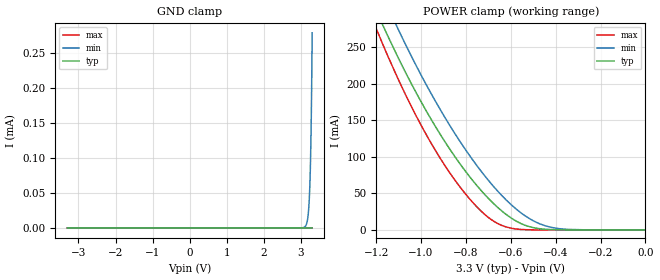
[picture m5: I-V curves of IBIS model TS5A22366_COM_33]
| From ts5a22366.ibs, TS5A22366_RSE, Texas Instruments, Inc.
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[Model]   TS5A22366_COM_33
Model_type  Terminator
| variable   typ   min   max
C_comp   111.30pF   73.64pF   137.43pF
| C_tri-state   111.30pF   73.64pF   137.43pF
[Temperature Range]   40   100   -40
| Ambient temperature   25   85   -40
[Voltage range]   3.3   3   3.6
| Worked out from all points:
|   POWER clamp passes 1 mA (typ) near -0.45 V on its own axis
[GND Clamp]
| TS5A22366_COM_33
|   Voltage   I(typ)   I(min)   I(max)
-3.3V     -7.249nA   -333.8nA   -3.915nA
3.1V      3.718nA    1.468uA    3.133nA
3.15V     3.782nA    5.921uA    3.187nA
3.185V    3.83nA     15.41uA    3.225nA
3.21V     3.87nA     29.93uA    3.251nA
3.235V    3.925nA    57.05uA    3.278nA
3.255V    3.995nA    94.24uA    3.3nA
3.27V     4.079nA    136.2uA    3.316nA
3.28V     4.162nA    173.4uA    3.327nA
3.285V    4.215nA    195.4uA    3.332nA
3.295V    4.353nA    247.6uA    3.343nA
3.3V      4.444nA    278.4uA    3.348nA
[POWER Clamp]
| TS5A22366_COM_33
|   Voltage   I(typ)   I(min)   I(max)
-3.3V     2.841A     2.858A     3.14A
-1.21V    307.7mA    348.5mA    283.5mA
-1.19V    293.8mA    334.3mA    268.5mA
-1.165V   276.8mA    316.9mA    250.3mA
-1.105V   237.9mA    276.9mA    208.7mA
-995mV    173mA      209.4mA    140.7mA
-870mV    109.8mA    142.2mA    77.4mA
-770mV    67.82mA    96.05mA    37.86mA
-670mV    34.19mA    57.2mA     10.84mA
-555mV    8.821mA    23.49mA    730.7uA
-445mV    913.3uA    5.582mA    18.08uA
0V        0A         0A         0A
